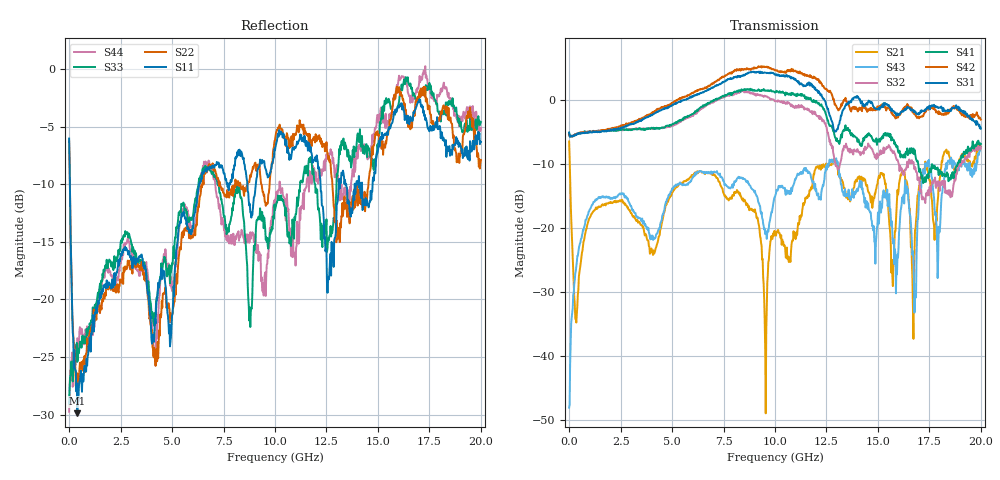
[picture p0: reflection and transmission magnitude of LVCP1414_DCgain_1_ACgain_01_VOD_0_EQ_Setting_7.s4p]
!Agilent Technologies,N5230A,MY46400459,A.07.50.48
!Agilent N5230A: A.07.50.48
!Date: Tuesday, April 17, 2012 18:47:18
!Correction: S11(Full 4 Port(1,2,3,4))
!S12(Full 4 Port(1,2,3,4))
!S13(Full 4 Port(1,2,3,4))
!S14(Full 4 Port(1,2,3,4))
!S21(Full 4 Port(1,2,3,4))
!S22(Full 4 Port(1,2,3,4))
!S23(Full 4 Port(1,2,3,4))
!S24(Full 4 Port(1,2,3,4))
!S31(Full 4 Port(1,2,3,4))
!S32(Full 4 Port(1,2,3,4))
!S33(Full 4 Port(1,2,3,4))
!S34(Full 4 Port(1,2,3,4))
!S41(Full 4 Port(1,2,3,4))
!S42(Full 4 Port(1,2,3,4))
!S43(Full 4 Port(1,2,3,4))
!S44(Full 4 Port(1,2,3,4))
!S4P File: Measurements: <S11,S12,S13,S14>,
!<S21,S22,S23,S24>,
!<S31,S32,S33,S34>,
!<S41,S42,S43,S44>:
# Hz S  dB  R 50
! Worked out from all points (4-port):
!   801 points, 300 kHz to 20 GHz, reference 50 ohm
!   strongest paths, dB at 300 kHz, 5 GHz, 10 GHz, 15 GHz, 20 GHz:
!     S31: -5.0, -0.8, 4.0, -1.4, -4.4
!     S42: -5.3, -0.4, 4.7, -1.0, -3.0
!     S41: -5.1, -3.7, 1.2, -6.2, -6.8
!     S32: -5.3, -4.0, -0.2, -8.9, -7.5
!     S43: -48.0, -13.8, -15.1, -17.5, -7.4
!     S21: -6.4, -14.4, -21.0, -12.5, -7.2
!   lowest |S11| = -29.9 dB at 400.3 MHz (marker M1), VSWR 1.07, Z = 53 + j1.29 ohm
!   |S11| at or under -10 dB: 37.28 MHz to 6.317 GHz (6.28 GHz wide, 198 % of centre); 12.21 GHz to 13.11 GHz (894.9 MHz wide, 7.07 % of centre); 14.23 GHz to 14.74 GHz (514.5 MHz wide, 3.55 % of centre)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
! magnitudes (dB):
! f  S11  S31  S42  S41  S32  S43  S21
! 300 kHz  -6.0  -5.0  -5.3  -5.1  -5.3  -48.0  -6.4
! 400.3 MHz  -29.9  -5.2  -5.2  -5.2  -5.2  -24.3  -32.1
! 9.95 GHz  -7.7  4.2  4.8  1.4  0.1  -15.5  -21.2
! 12.88 GHz  -14.9  -4.7  -0.2  -5.3  -8.9  -9.3  -9.5
! 14.03 GHz  -10.0  0.5  -1.7  -6.5  -8.0  -14.2  -12.0
! 16.78 GHz  -3.7  -1.6  -2.1  -7.7  -10.8  -33.2  -24.0
! 20 GHz  -6.3  -4.4  -3.0  -6.8  -7.5  -7.4  -7.2
